|//////////////////////////////////////////////////////////////////////////////
|//////////////////////////////////////////////////////////////////////////////
|   @@@@@@@   @@@@@@@   @@@@@@@   @@@@@@@   @@@@@@@   @@@@@@   @@
|   @@@@@@@@@   @@@@@@@@@   @@@@@@@@@   @@@@@@@@@   @@@@@@@@@ @@@@@@@@  @
|   @@@   @@@ @@@   @@@ @@@   @@@   @@@ @@@   @@@@   @@@  @
|   @@   @@ @@   @@ @@@@@@@@@@@ @@@@@@@@@@@ @@   @@   @@ @@
|   @@@   @@@ @@   @@   @@@ @@@   @@   @@   @@ @@
|   @@@@@@@@@  @@   @@  @@@@@@@@@   @@@@@@@@@  @@   @@   @@ @@
|   @@@@@@@   @@   @@   @@@@@@@   @@@@@@@   @@   @@   @@ @@
|   IBIS Model of NL3V1T34
|   1-Bit Dual-Supply Level Translator
|   Package Type: UDFN6, CASE 517AQ  (1.45 x 1.00 mm)
|   UDFN6, CASE 517AA  (1.20 x 1.00 mm)
|   SC-88A (SOT-353/SC-70-5), CASE 419A-02
|   The model is covering the following Vccs:
|   0.9V, 1.2V, 1.5V, 1.8V, 2.5V, 3.3V
|//////////////////////////////////////////////////////////////////////////////
|//////////////////////////////////////////////////////////////////////////////
[IBIS Ver]   3.2
|   7.2 compatible
|//////////////////////////////////////////////////////////////////////////////
[Comment Char] |_char
|//////////////////////////////////////////////////////////////////////////////
[File Name]   nl3v1t34_va_r0.ibs
|//////////////////////////////////////////////////////////////////////////////
[File Rev]   0.0
|   0.0 - May 23, 2025 - File created
|//////////////////////////////////////////////////////////////////////////////
[Date]   May 23, 2025
|//////////////////////////////////////////////////////////////////////////////
[Source]   From lab measurements and simulations at onsemi
|//////////////////////////////////////////////////////////////////////////////
[Notes]   - The currents greater than +/- 100 mA are extrapolated
|//////////////////////////////////////////////////////////////////////////////
[Disclaimer]
   - onsemi Corporation hereby grants
   the user of this IBIS model a license to use this model
   under the following terms. This license is nonexclusive
   and nontransferable. Before using this IBIS model.
   After reading the terms and conditions of this license,
   the user either must accept these terms,
   or the IBIS model should be returned to onsemi within 30 days.
   - The user is hereby granted a license to use the IBIS model.
   This shall not be construed as a right to sell,
   or otherwise profit either by leasing or renting this software.
   - The user may modify the IBIS model to suit his specific
   applications but rights to derivative works and such
   modifications shall belong to onsemi.
   - This IBIS model is provided on an "as is" basis.
   onsemi makes absolutely no warranty with respect
   to the information contained herein.
   By use of this IBIS model, the user assumes full risk as to the
   quality and suitablility of the model to his particular use,
   and by using this model assumes the entire risk.
   Under all circumstances the user shall not hold
   onsemi liable in any way for the results obtained.
   onsemi reserves the right to make to improve
   the model for reliability, function, or design.
   onsemi does not convey any license under patent
   rights or any other intellectual property rights,
   including those of third parties.
   - onsemi is not obligated to provide maintenance
   or support for the licensed IBIS model.
   - Cont onsemi at ATTN:LOGIC APPLICATIONS/IBIS MODEL.
   5701 N Pima Rd, Scottsdale, AZ 85250
|//////////////////////////////////////////////////////////////////////////////
[Copyright]   (c) 2025 onsemi Corp.
|//////////////////////////////////////////////////////////////////////////////
|//////////////////////////////////////////////////////////////////////////////
[Component]   NL3V1T34MU1TAG
|//////////////////////////////////////////////////////////////////////////////
[Manufacturer]  onsemi
|   Data Sheet: NL3V1T244/D, May, 2025 - Rev. P2
|//////////////////////////////////////////////////////////////////////////////
[Package]
|   UDFN-6
| 1.45 x 1.0
| CASE 517AQ
| variable   typ   min   max
R_pkg   0.0499   0.0010   0.0568
L_pkg   0.4063nH   0.0145nH   0.4786nH
C_pkg   0.1074pF   0.0765pF   0.1119pF
|//////////////////////////////////////////////////////////////////////////////
[Pin] signal_name   model_name   R_pin   L_pin   C_pin
1   VCCA   POWER   0.0568   0.4786nH   0.1119pF
2   A   In1   0.0469   0.3812nH   0.1077pF
3   GND   GND   0.0541   0.4521nH   0.1099pF
4   B   Out   0.0513   0.4206nH   0.1072pF
5   NC   NC   0.0010   0.0145nH   0.0765pF
6   VCCB   POWER   0.0484   0.3921nH   0.1051pF
|//////////////////////////////////////////////////////////////////////////////
|//////////////////////////////////////////////////////////////////////////////
[Component]   NL3V1T34MU1TCG
|//////////////////////////////////////////////////////////////////////////////
[Manufacturer]  onsemi
|   Data Sheet: NL3V1T244/D, May, 2025 - Rev. P2
|//////////////////////////////////////////////////////////////////////////////
[Package]
R_pkg   0.0499   0.0010   0.0568
L_pkg   0.4063nH   0.0145nH   0.4786nH
C_pkg   0.1074pF   0.0765pF   0.1119pF
|//////////////////////////////////////////////////////////////////////////////
[Pin] signal_name   model_name   R_pin   L_pin   C_pin
1   VCCA   POWER   0.0568   0.4786nH   0.1119pF
2   A   In1   0.0469   0.3812nH   0.1077pF
3   GND   GND   0.0541   0.4521nH   0.1099pF
4   B   Out   0.0513   0.4206nH   0.1072pF
5   NC   NC   0.0010   0.0145nH   0.0765pF
6   VCCB   POWER   0.0484   0.3921nH   0.1051pF
|//////////////////////////////////////////////////////////////////////////////
|//////////////////////////////////////////////////////////////////////////////
[Component]   NL3V1T34MU2TBG
|//////////////////////////////////////////////////////////////////////////////
[Manufacturer]  onsemi
|   Data Sheet: NL3V1T244/D, May, 2025 - Rev. P2
|//////////////////////////////////////////////////////////////////////////////
[Package]
|  UDFN-6
| 1.2 x 1.0
| CASE 517AA
| variable   typ   min   max
R_pkg   0.0380   0.0007   0.0502
L_pkg   0.3514nH   0.0262nH   0.4657nH
C_pkg   0.1033pF   0.0765pF   0.1113pF
|//////////////////////////////////////////////////////////////////////////////
[Pin] signal_name   model_name   R_pin   L_pin   C_pin
1   VCCA   POWER   0.0495   0.4460nH   0.1109pF
2   A   In1   0.0407   0.3641nH   0.1069pF
3   GND   GND   0.0492   0.4551nH   0.1110pF
4   B   Out   0.0502   0.4657nH   0.1113pF
5   NC   NC   0.0007   0.0262nH   0.0765pF
6   VCCB   POWER   0.0461   0.4205nH   0.1085pF
|//////////////////////////////////////////////////////////////////////////////
|//////////////////////////////////////////////////////////////////////////////
[Component]   NL3V1T34DFT2G
|//////////////////////////////////////////////////////////////////////////////
[Manufacturer]  onsemi
|   Data Sheet: NL3V1T244/D, May, 2025 - Rev. P2
|//////////////////////////////////////////////////////////////////////////////
[Package]
| SC-88A / SC-70-5
|   DF SUFFIX
|   CASE 419A-02
| variable   typ   min   max
R_pkg   0.0201   0.0170   0.0250
L_pkg   0.9982nH   0.8810nH   1.0690nH
C_pkg   0.1466pF   0.1187pF   0.2051pF
|//////////////////////////////////////////////////////////////////////////////
[Pin] signal_name   model_name   R_pin   L_pin   C_pin
1   VCCA   POWER   0.0191   1.0690nH   0.1625pF
2   A   In1   0.0187   0.8810nH   0.1217pF
3   GND   GND   0.0170   1.0315nH   0.2051pF
4   B   Out   0.0207   0.9600nH   0.1249pF
5   VCCB   POWER   0.0250   1.0497nH   0.1187pF
|//////////////////////////////////////////////////////////////////////////////
|//////////////////////////////////////////////////////////////////////////////
[Component]   NL3V1T34DFT2G-Q
|//////////////////////////////////////////////////////////////////////////////
[Manufacturer]  onsemi
|   Data Sheet: NL3V1T244/D, May, 2025 - Rev. P2
|//////////////////////////////////////////////////////////////////////////////
[Package]
R_pkg   0.0201   0.0170   0.0250
L_pkg   0.9982nH   0.8810nH   1.0690nH
C_pkg   0.1466pF   0.1187pF   0.2051pF
|//////////////////////////////////////////////////////////////////////////////
[Pin] signal_name   model_name   R_pin   L_pin   C_pin
1   VCCA   POWER   0.0191   1.0690nH   0.1625pF
2   A   In1   0.0187   0.8810nH   0.1217pF
3   GND   GND   0.0170   1.0315nH   0.2051pF
4   B   Out   0.0207   0.9600nH   0.1249pF
5   VCCB   POWER   0.0250   1.0497nH   0.1187pF |
|//////////////////////////////////////////////////////////////////////////////
|//////////////////////////////////////////////////////////////////////////////
[Model Selector]   In1
In1_09   Vcc = 0.90
In1_12   Vcc = 1.20
In1_15   Vcc = 1.50
In1_18   Vcc = 1.80
In1_25   Vcc = 2.50
In1_33   Vcc = 3.30
|//////////////////////////////////////////////////////////////////////////////
[Model Selector]   In2
In2_09   Vcc = 0.90
In2_12   Vcc = 1.20
In2_15   Vcc = 1.50
In2_18   Vcc = 1.80
In2_25   Vcc = 2.50
In2_33   Vcc = 3.30
|//////////////////////////////////////////////////////////////////////////////
[Model Selector]   Out
Out_09   Vcc = 0.90
Out_12   Vcc = 1.20
Out_15   Vcc = 1.50
Out_18   Vcc = 1.80
Out_25   Vcc = 2.50
Out_33   Vcc = 3.30
| Models and submodels in the file (18): In1_09 (Input), In2_09 (Input), Out_09 (3-state), In1_12 (Input), In2_12 (Input), Out_12 (3-state), In1_15 (Input), In2_15 (Input), Out_15 (3-state), In1_18 (Input), In2_18 (Input), Out_18 (3-state), In1_25 (Input), In2_25 (Input), Out_25 (3-state), In1_33 (Input), In2_33 (Input), Out_33 (3-state)
